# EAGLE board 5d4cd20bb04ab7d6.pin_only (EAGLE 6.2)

Size 30.48 x 30.48 mm. Coordinates in mm from the lower left corner, seen from the top.
Outline: 15.24,0 arc-90 0,15.24 arc-90 15.24,30.48 arc-90 30.48,15.24 arc-90 15.24,0
Copper layers (1*16): Top 0.035mm / dielectric 1.5mm / Bottom 0.035mm
Design rules: minimum track width 8mil, minimum drill 0.4mm, track to track 8mil, track to pad 8mil, pad to pad 8mil, via to via 8mil, smd to smd 8mil, copper to edge 20mil, drill to drill 8mil, minimum pad ring 8mil, minimum via ring 10mil, stop-mask expansion 3mil, vias tented up to drill 20mil, thermal gap 8mil

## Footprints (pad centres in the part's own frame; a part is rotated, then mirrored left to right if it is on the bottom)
SEWINGTAP_2.0 = drill 1.5 pad 2.54: P$1 0,0
0805 = smd 1.3 x 1.5: 1 -0.95,0; 2 0.95,0
FIDUCIAL_1MM = smd 1 x 1: 1 0,0
CHIPLED_0805 = smd 1.2 x 1.2: A 0,-1.05; C 0,1.05
FGPMMOPA6H = smd 2 x 1: P$1 -7.5,6.75; P$2 -7.5,5.25; P$3 -7.5,3.75; P$4 -7.5,2.25; P$5 -7.5,0.75; P$6 -7.5,-0.75; P$7 -7.5,-2.25; P$8 -7.5,-3.75; P$9 -7.5,-5.25; P$10 -7.5,-6.75; P$11 7.5,-6.75; P$12 7.5,-5.25; P$13 7.5,-3.75; P$14 7.5,-2.25; P$15 7.5,-0.75; P$16 7.5,0.75; P$17 7.5,2.25; P$18 7.5,3.75; P$19 7.5,5.25; P$20 7.5,6.75 | hole 3: 0.5,0.85
U.FL = smd 2.2 x 0.85: P$1 0,1.375; P$2 0,-1.375 | smd 1.05 x 1: P$3 1.525,0; P$4 -1.525,0

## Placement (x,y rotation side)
3V3IN  SEWTAP-2.0IN  [SEWINGTAP_2.0]  26.92,10.54 247.5 top
C2  10uF  [0805]  15.26,4.83 180 top
FB1  Ferrite  [0805]  24.28,6.06 225 top
FID1  FIDUCIAL""  [FIDUCIAL_1MM]  20.19,19.05 0 top
FID2  FIDUCIAL""  [FIDUCIAL_1MM]  9.42,11.47 0 top
GND  SEWTAP-2.0IN  [SEWINGTAP_2.0]  3.56,10.54 112.5 top
GND1  SEWTAP-2.0IN  [SEWINGTAP_2.0]  10.41,26.8 22.5 top
LED1  FIX  [CHIPLED_0805]  26.82,17.65 180 top
R1  1K  [0805]  24.79,17.65 270 top
RX  SEWTAP-2.0IN  [SEWINGTAP_2.0]  10.41,3.68 157.5 top
TP1  SEWTAP-2.0IN  [SEWINGTAP_2.0]  3.56,19.94 67.5 top
TP4  SEWTAP-2.0IN  [SEWINGTAP_2.0]  20.07,26.8 337.5 top
TX  SEWTAP-2.0IN  [SEWINGTAP_2.0]  20.07,3.68 202.5 top
U1  FGPMMOPA6H  [FGPMMOPA6H]  15.24,15.24 90 top
U$6  [ADAFRUIT_5MM]  12.83,24 0 top
U$7  [FLORASMALL]  24.77,22.99 270 bottom
U$20  U.FL  [U.FL]  25.65,22.35 180 top

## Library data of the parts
3V3IN GND GND1 RX TP1 TP4 TX = adafruit
C2 FB1 FID1 FID2 LED1 R1 U1 U$6 U$20 = microbuilder
U$7 = flora

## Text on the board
tPlace: GND | FIX | BAT | GND | 3.3V | RX | TX
bDocu: Flora GPS Module | 3.3V @ 20-25mA | Version 1.0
